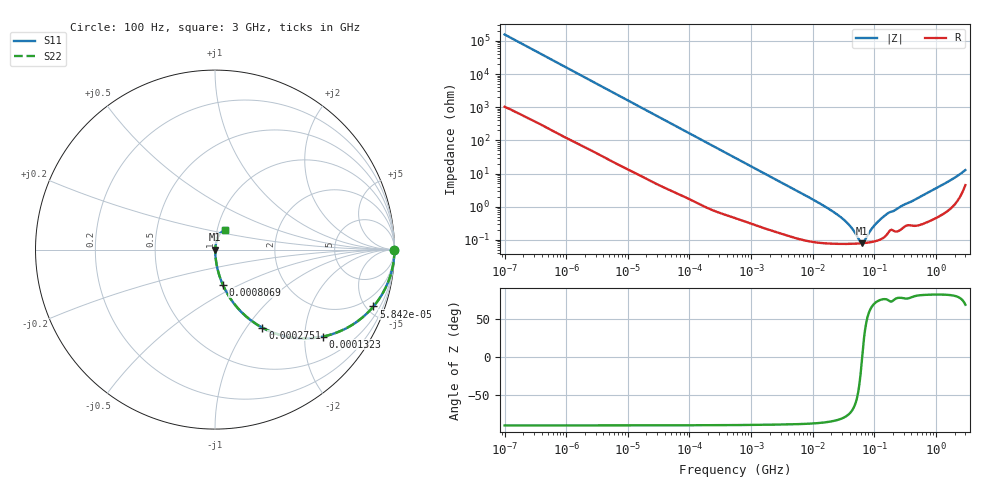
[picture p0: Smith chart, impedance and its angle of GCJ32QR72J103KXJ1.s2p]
!Murata Part Number: GCJ32QR72J103KXJ1
!These Parameters are Measured in Series Mode Connection
!Data Generated on Mar 13, 2026
!  o--ll--o
!Port1  Port2
!  o------o
!Operation Temp=25[degC], DC Bias Voltage=0[V]
!Freq. Start=100[Hz] Stop=3[GHz] 401[Steps]
# Hz S RI R 50
!Freq.(Hz) S11(Real) S11(Imag) S21(Real) S21(Imag) S12(Real) S12(Imag) S22(Real) S22(Imag)
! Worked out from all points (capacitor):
!   401 points, 100 Hz to 3 GHz, reference 50 ohm
!   read as one part in series: C = 10.1 nF near 109 Hz
!   lowest |Z| = 78.9 mohm at 62.34 MHz (marker M1)
!   series resonance near 63.34 MHz, so ESL is about 620 pH
!   S11 on the Smith chart (normalised r, x): 100 Hz: open; 58.42 kHz: 1.05, -5.55; 132.3 kHz: 1.03, -2.46; 275.1 kHz: 1.01, -1.19; 806.9 kHz: 1.01, -0.41; 3 GHz: 1.09, +0.24
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100  1 -0.000637  4.6e-06 0.000637  4.6e-06 0.000637  1 -0.000637
1788  0.9998 -0.0112  0.000214 0.0112  0.000214 0.0112  0.9998 -0.0112
10003  0.9956 -0.062  0.00437 0.062  0.00437 0.062  0.9956 -0.062
31977  0.9608 -0.1898  0.0392 0.1898  0.0392 0.1898  0.9608 -0.1898
58416  0.8828 -0.3169  0.1172 0.3169  0.1172 0.3169  0.8828 -0.3169
132342  0.6017 -0.4843  0.3983 0.4843  0.3983 0.4843  0.6017 -0.4843
275091  0.2639 -0.4349  0.7361 0.4349  0.7361 0.4349  0.2639 -0.4349
547723  0.0861 -0.2731  0.9139 0.2731  0.9139 0.2731  0.0861 -0.2731
806856  0.0432 -0.195  0.9568 0.195  0.9568 0.195  0.0432 -0.195
2266852  0.00717 -0.0728  0.9928 0.0728  0.9928 0.0728  0.00717 -0.0728
9794414  0.00115 -0.0168  0.9989 0.0168  0.9989 0.0168  0.00115 -0.0168
1.950129e7  0.000826 -0.00786  0.9992 0.00786  0.9992 0.00786  0.000826 -0.00786
3.131008e7  0.000766 -0.00409  0.9992 0.00409  0.9992 0.00409  0.000766 -0.00409
4.231884e7  0.00076 -0.00222  0.9992 0.00222  0.9992 0.00222  0.00076 -0.00222
5.719833e7  0.000775 -0.000547  0.9992 0.000547  0.9992 0.000547  0.000775 -0.000547
6.234031e7  0.000784 -8.4e-05  0.9992 8.4e-05  0.9992 8.4e-05  0.000784 -8.4e-05
6.794454e7  0.000796 0.000379  0.9992 -0.000379  0.9992 -0.000379  0.000796 0.000379
8.79653e7  0.000851 0.0018  0.9991 -0.0018  0.9991 -0.0018  0.000851 0.0018
1.090876e8  0.000939 0.00309  0.9991 -0.00309  0.9991 -0.00309  0.000939 0.00309
1.751444e8  0.00185 0.00644  0.9981 -0.00644  0.9981 -0.00644  0.00185 0.00644
1.268426e9  0.00774 0.0445  0.9923 -0.0445  0.9923 -0.0445  0.00774 0.0445
3e9  0.0551 0.1076  0.9449 -0.1076  0.9449 -0.1076  0.0551 0.1076
